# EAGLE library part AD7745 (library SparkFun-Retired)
24-bit capacitance to digital converter Not in catalog
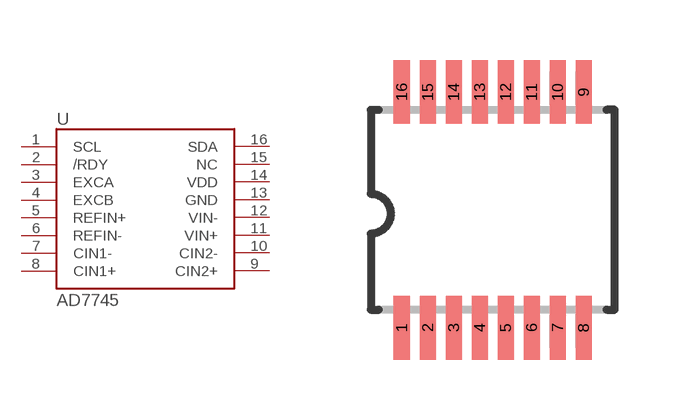
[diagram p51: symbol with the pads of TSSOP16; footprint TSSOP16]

Designator prefix -

## AD7745  [TSSOP16]
1  SCL
2  /RDY
3  EXCA
4  EXCB
5  REFIN+
6  REFIN-
7  CIN1-
8  CIN1+
9  CIN2+
10  CIN2-
11  VIN+
12  VIN-
13  GND
14  VDD
15  NC
16  SDA

## Footprint TSSOP16 (pad centres in mm)
TSOP16 thin small outline package
smd 0.4 x 1.6: 1 -2.225,-2.85; 2 -1.575,-2.85; 3 -0.925,-2.85; 4 -0.275,-2.85; 5 0.375,-2.85; 6 1.025,-2.85; 7 1.675,-2.85; 8 2.325,-2.85; 9 2.325,3.05; 10 1.675,3.05; 11 1.025,3.05; 12 0.375,3.05; 13 -0.275,3.05; 14 -0.925,3.05; 15 -1.575,3.05; 16 -2.225,3.05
